FUNCTION_BLOCK FB_Base EXTENDS FB_BasePart IMPLEMENTS I_Elementinformation, I_TestInterface
(*
 @details
 The FB_Base is the base function block of the.
 @usage
 The function block works like this or like that.
 also there are multiline stuff possible
*)
VAR
	//Elementinformation
  _bCodeActive 						: BOOL; // this does that or those
	_bEnableCode              			: BOOL;  (* other possible comment *)          

	{attribute 'hide'}                							
	_bUseParentEnableCode				: BOOL; (*** other possible comment *)
	
    _bEnableAlarm         				: BOOL := TRUE;
    {attribute 'hide'}
	_bUseParentEnableAlarm				: BOOL;   
		
    _eSimulation      					: E_SimulationMode := E_SimulationMode.simOff;
    {attribute 'hide'}
	_bUseParentSimulation				: BOOL;
	
	_bReset								: BOOL;
    {attribute 'hide'}
	_bUseParentReset					: BOOL;
	
	_nParentNumber						: INT;
    {attribute 'hide'}
	_bUseParentNumber					: BOOL;
	
	_sParentName						: STRING(Par_Core.C_nLengthOfParentName);
    {attribute 'hide'}
	_bUseParentName						: BOOL;	
	
    _sDesignationName     				: STRING(Par_Core.C_nLengthOfDesignationName);      
	
	_bError								: BOOL;
	
    {attribute 'hide'}
    _iParentInformation 				: I_ElementInformation;												
    {attribute 'hide'}
    _eCodeExecution 					: E_CodeExecutionMode; 										
	
	// Logging
	{attribute 'hide'}
	_LogCollector						: FB_LogCollector;
    {attribute 'hide'}	        		
	_BaseLogger							: FB_Log := (logCollector := _LogCollector);
END_VAR

VAR_STAT
	{attribute 'hide'}
	_bLicenseOk 							: BOOL := TRUE; // static class variable, access to all fb
END_VAR

METHOD PROTECTED _ConfigureAlarm : BOOL;
(***********************************************************************************
* @brief Description : Gets called in enabling
* @return None
************************************************************************************)
// Call update once to enable/disableAlarms
_UpdateAlarm();
_BaseLogger.Info(sMsg := 'Alarms configured').Send();
_ConfigureAlarm := TRUE;
END_METHOD

METHOD PROTECTED _ConfigureHmi : BOOL;
// gets called in enabling
// do some elementmgr magic
_BaseLogger.Debug(sMsg := 'HMI configured').Send();
_ConfigureHmi := TRUE;
END_METHOD

METHOD PROTECTED _Disabling : BOOL;
(***********************************************************************************
* @brief Description : Logic which disables the function block
* @return BOOL 1 = Disabling completed
************************************************************************************)
_ResetError(); // call reset method
_Disabling := _ConfigureAlarm() AND _ConfigureHmi();
END_METHOD

METHOD PROTECTED _Enabling : BOOL
_ResetError(); // call reset method
_Enabling := _ConfigureAlarm() AND _ConfigureHmi();
END_METHOD

METHOD PRIVATE _GetParentInformation
IF _iParentInformation <> 0 THEN
	IF _bUseParentEnableAlarm 	THEN _bEnableAlarm 		:= _iParentInformation.EnableAlarm; 	END_IF
	IF _bUseParentEnableCode 	THEN _bEnableCode 		:= _iParentInformation.EnableCode; 		END_IF
	IF _bUseParentReset 		THEN _bReset 			:= _iParentInformation.Reset; 			END_IF
	IF _bUseParentSimulation 	THEN _eSimulation 		:= _iParentInformation.Simulation; 		END_IF
	IF _bUseParentName 	THEN _sParentName 		:= _iParentInformation.ParentName; 		END_IF
	IF _bUseParentNumber 	THEN _nParentNumber 	:= _iParentInformation.ParentNumber; 	END_IF
END_IF
END_METHOD

METHOD PROTECTED _MainGeneral






_UpdateAlarm();
_UpdateHmi();
IF _bReset THEN
	_ResetError();
END_IF
END_METHOD

METHOD PROTECTED _ResetError
(***********************************************************************************
* @brief Description : Gets called if bReset is true, in enabling,disabling and maingeneral
* @return None
************************************************************************************)
// do some things








_UpdateAlarm();
_BaseLogger.Debug(sMsg := 'Reset triggered').Send();
END_METHOD

METHOD PROTECTED _SetError
(***********************************************************************************
* @brief Description : gets called by update Alarm, used to set the error bit
* @return None
************************************************************************************)
// set the function block error bit
_bError := FALSE;
END_METHOD

METHOD PROTECTED _UpdateAlarm
(***********************************************************************************
* @brief Description : Call of all alarm function blocks
* @return None
************************************************************************************)
//// Example







// Call error collection method
_SetError();
END_METHOD

METHOD PROTECTED _UpdateHmi
(***********************************************************************************
* @brief Description : Method to update the HMI interface
* @return None
************************************************************************************)
// copy all internal parameters to the HMI interface
END_METHOD

METHOD PUBLIC CyclicGeneral

VAR_INST
	{attribute 'hide'}
	_EnableCodeLogger 		: FB_LogVar := (LogCollector := LogCollector);
	{attribute 'hide'}
	_EnableAlarmLogger 		: FB_LogVar := (LogCollector := LogCollector);
	{attribute 'hide'}
	_CodeActiveLogger 		: FB_LogVar := (LogCollector := LogCollector);
	{attribute 'hide'}
	_DesignationNameLogger 	: FB_LogVar := (LogCollector := LogCollector);
	{attribute 'hide'}
	_SimulationLogger 		: FB_LogVar := (LogCollector := LogCollector);
	{attribute 'hide'}
	_ParentNameLogger 		: FB_LogVar := (LogCollector := LogCollector);
	{attribute 'hide'}
	_ParentNumberLogger 	: FB_LogVar := (LogCollector := LogCollector);
END_VAR
_GetParentInformation();
_EnableCodeLogger.OnChange(_bEnableCode);

CASE _eCodeExecution OF
    E_CodeExecutionMode.enable:
        IF _Enabling() THEN
            _eCodeExecution := E_CodeExecutionMode.cyclic;
        END_IF

    E_CodeExecutionMode.cyclic:
        IF NOT _bEnableCode OR NOT _bLicenseOk THEN
            _eCodeExecution := E_CodeExecutionMode.disable;
        END_IF

    E_CodeExecutionMode.disable:
        IF _Disabling() THEN
            _eCodeExecution := E_CodeExecutionMode.undefined;
        END_IF

    E_CodeExecutionMode.undefined:
        IF _bEnableCode AND _bLicenseOk THEN		
            _eCodeExecution := E_CodeExecutionMode.enable;
        END_IF
END_CASE

_bCodeActive := _eCodeExecution = E_CodeExecutionMode.cyclic;
_CodeActiveLogger.OnChange(_bCodeActive);

IF _bCodeActive THEN
	_DesignationNameLogger.OnChange(_sDesignationName);
	_ParentNameLogger.OnChange(_sParentName);
	_ParentNumberLogger.OnChange(_nParentNumber);
	_EnableAlarmLogger.OnChange(_bEnableCode);
	_SimulationLogger.OnChange(_eSimulation);
    _MainGeneral();
END_IF
END_METHOD

PROPERTY DesignationName : String(Par_Core.C_nLengthOfDesignationName)
GET
DesignationName := THIS^._sDesignationName;
END_GET
SET
THIS^._sDesignationName := DesignationName;
END_SET
END_PROPERTY

PROPERTY EnableAlarm : BOOL
GET
EnableAlarm := THIS^._bEnableAlarm;
END_GET
SET
_bUseParentEnableAlarm := FALSE;
THIS^._bEnableAlarm := EnableAlarm;
END_SET
END_PROPERTY

PROPERTY EnableCode : Bool
GET
EnableCode := THIS^._bCodeActive;
END_GET
SET
_bUseParentEnableCode := FALSE;
THIS^._bEnableCode := EnableCode;
END_SET
END_PROPERTY

PROPERTY Error : BOOL
GET
Error := THIS^._bError;
END_GET
END_PROPERTY

PROPERTY LogCollector : REFERENCE TO FB_LogCollector
GET
LogCollector REF= _LogCollector;
END_GET
END_PROPERTY

PROPERTY Parent : I_ElementInformation
SET
_iParentInformation 			:= Parent;
// Reset all information selectors
_bUseParentReset 			:= TRUE;
_bUseParentEnableCode 		:= TRUE;
_bUseParentEnableAlarm 		:= TRUE;
_bUseParentSimulation 		:= TRUE;
_bUseParentNumber		:= TRUE;
_bUseParentName		:= True;
END_SET
END_PROPERTY

PROPERTY ParentName : STRING(Par_Core.C_nLengthOfParentName)
GET
ParentName := THIS^._sParentName;
END_GET
SET
_bUseParentName := FALSE;
THIS^._sParentName := ParentName;
END_SET
END_PROPERTY

PROPERTY ParentNumber : INT
GET
ParentNumber := THIS^._nParentNumber;
END_GET
SET
_bUseParentNumber := FALSE;
THIS^._nParentNumber := ParentNumber;
END_SET
END_PROPERTY

PROPERTY Reset : BOOL
GET
Reset := THIS^._bReset;
END_GET
SET
_bUseParentReset := FALSE;
THIS^._bReset := Reset;
END_SET
END_PROPERTY

PROPERTY Simulation : E_SimulationMode
GET
Simulation := THIS^._eSimulation;
END_GET
SET
_bUseParentSimulation := FALSE;
THIS^._eSimulation := Simulation;
END_SET
END_PROPERTY

END_FUNCTION_BLOCK
